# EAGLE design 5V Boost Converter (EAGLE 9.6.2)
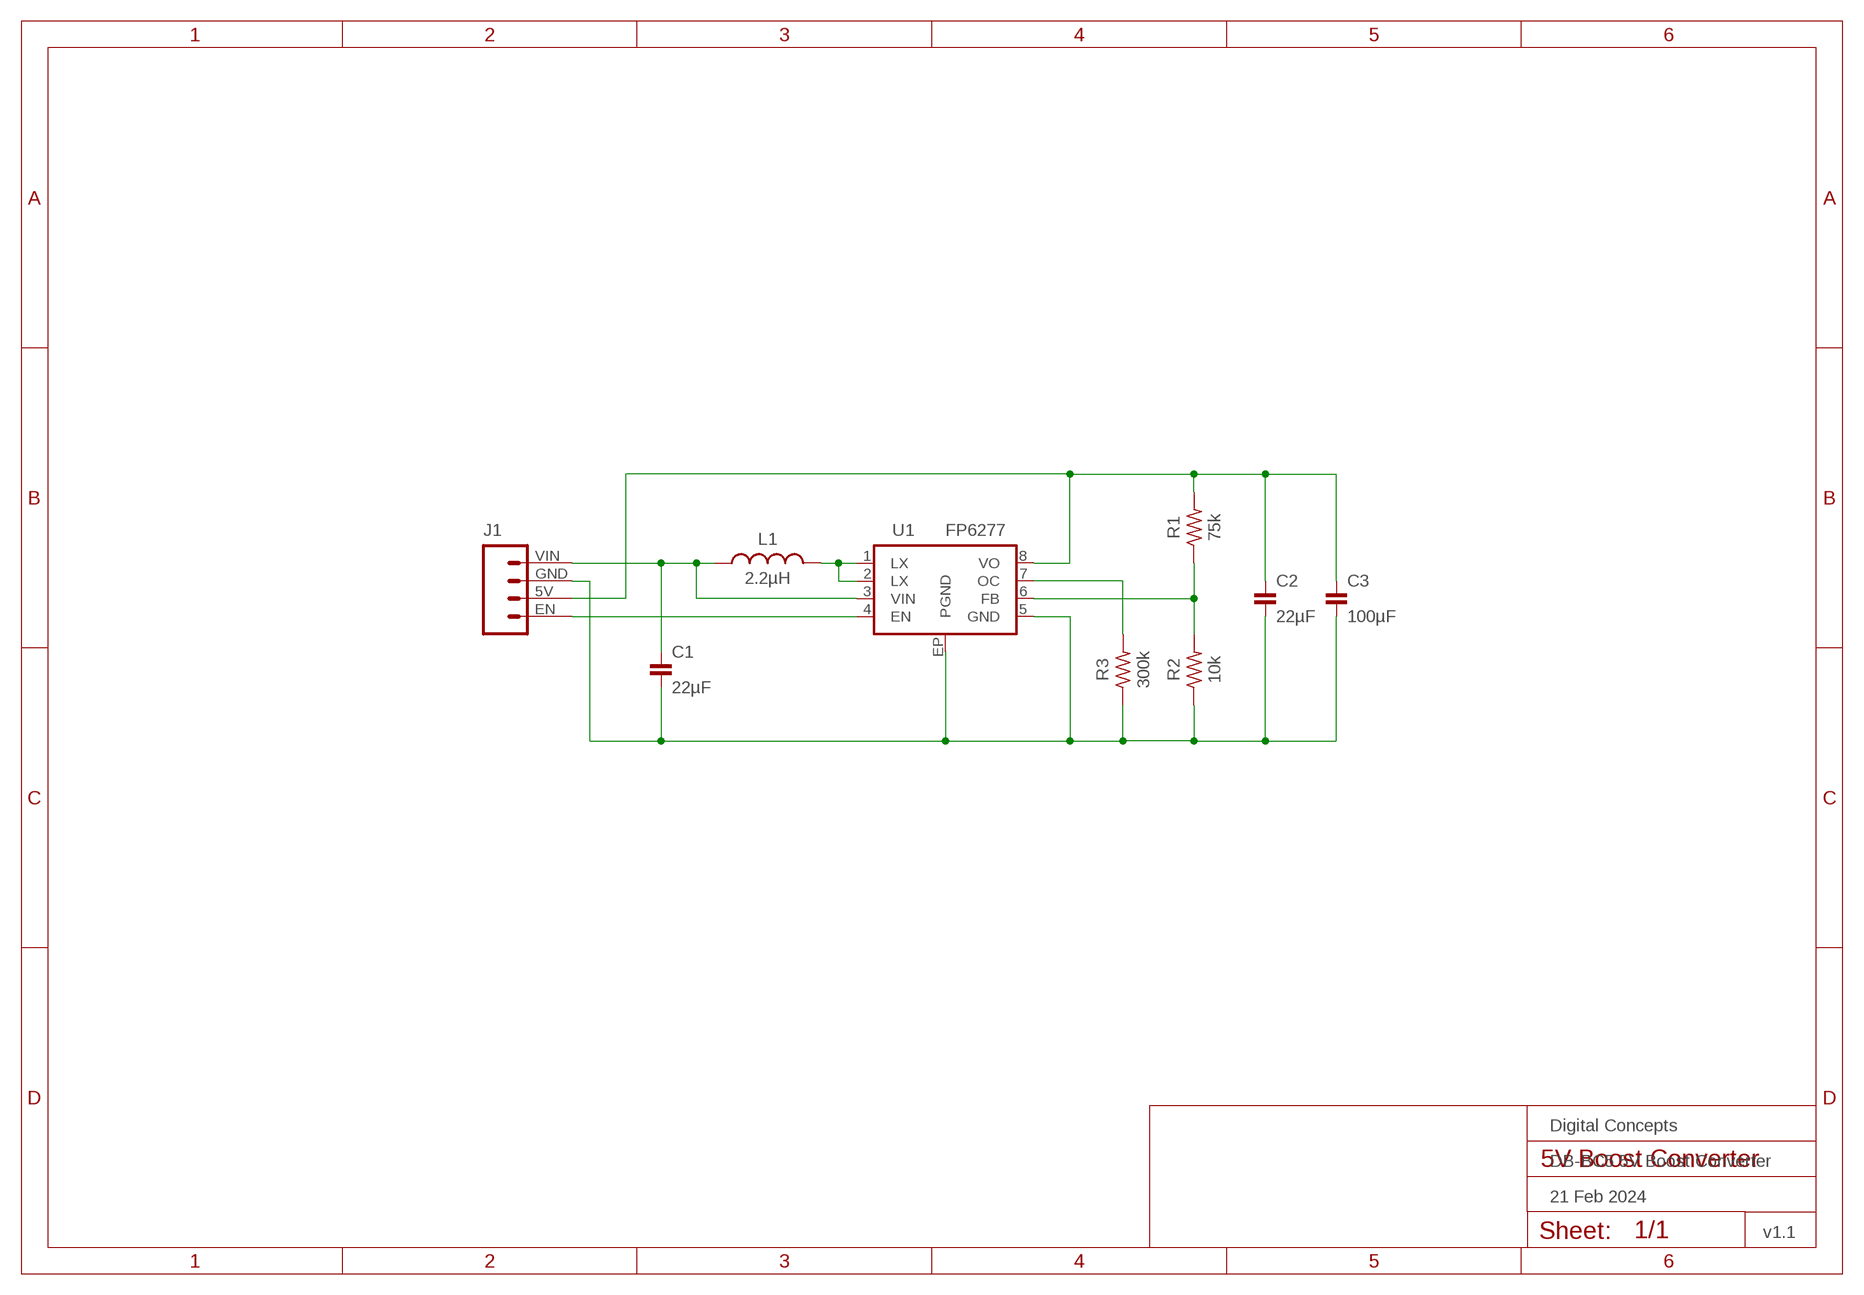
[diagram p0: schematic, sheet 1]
FRAME2 (FRAME-A4L-LOC): DATE: 21 Feb 2024; OWNER: Digital Concepts; TITLE: DB-BC5 5V Boost Converter; VERSION: v1.1

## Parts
C1  22µF  CAPACITOR-0805  [C0805]
C2  22µF  CAPACITOR-0805  [C0805]
C3  100µF  CAPACITOR-1206  [C1206]
J1  HEADER-1X4-FP6277  [CONN_04-FP6277]
L1  2.2µH  INDUCTOR-LQM2HPN2R2MG0L  [L1008]
R1  75k  RESISTORR0805  [R0805]
R2  10k  RESISTORR0805  [R0805]
R3  300k  RESISTORR0805  [R0805]
U1  FP6277  [SOP-8(EP)]

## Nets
5V: C2.1 C3.1 J1.5V R1.2 U1.8(VO)
EN: J1.EN U1.4(EN)
GND: C1.2 C2.2 C3.2 J1.GND R2.1 R3.1 U1.5(GND) U1.EP(PGND)
N$2: L1.P$1 U1.1(LX) U1.2(LX)
N$3: R1.1 R2.2 U1.6(FB)
N$5: R3.2 U1.7(OC)
VIN: C1.1 J1.VIN L1.P$2 U1.3(VIN)

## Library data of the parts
C1 C2 = digitalconcepts:CAPACITOR-0805: 0805 Capacitor
C3 = digitalconcepts:CAPACITOR-1206: 1206 Capacitor
J1 = digitalconcepts:HEADER-1X4-FP6277: FP6277 4-Pin Header
L1 = digitalconcepts:INDUCTOR-LQM2HPN2R2MG0L: LQM2HPN2R2MG0L
R1-R3 = digitalconcepts:RESISTOR: Resistor; SPICEPREFIX: R
U1 = digitalconcepts:FP6277: FP6277 Boost Controller

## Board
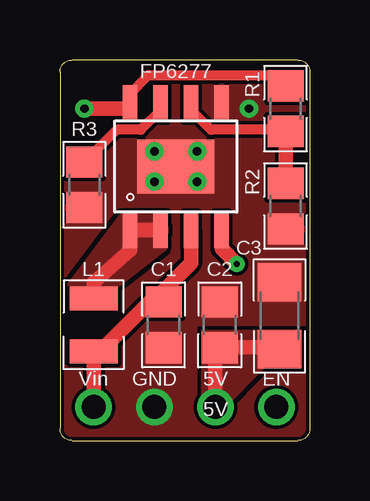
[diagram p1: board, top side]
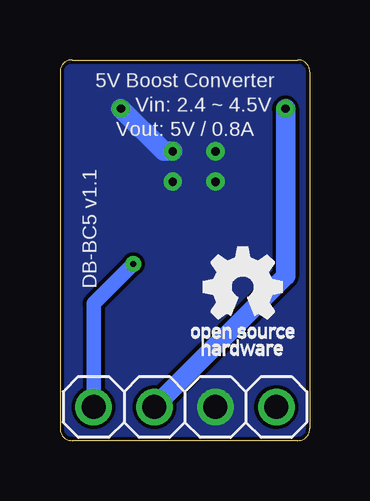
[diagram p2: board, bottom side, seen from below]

Size 10.41 x 15.88 mm. Coordinates in mm from the lower left corner, seen from the top.
Outline: 9.91,15.88 arc-90 10.41,15.37 10.41,0.51 arc-90 9.91,0 0.51,0 arc-90 0,0.51 0,15.37 arc-90 0.51,15.88 9.91,15.88
Copper layers (1*16): Top 0.035mm / dielectric 1.5mm / Bottom 0.035mm
Design rules "default *": minimum track width 6mil, minimum drill 0.15mm, track to track 6mil, track to pad 6mil, pad to pad 6mil, via to via 6mil, smd to smd 6mil, copper to edge 6mil, drill to drill 6mil, minimum pad ring 10mil, minimum via ring 8mil, stop-mask expansion 4mil, vias tented up to drill 0mil, thermal gap 0mil

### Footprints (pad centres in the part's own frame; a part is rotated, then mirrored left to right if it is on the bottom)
C0805 = smd 1.3 x 1.5: 1 -0.95,0; 2 0.95,0
C1206 = smd 1.6 x 1.8: 1 -1.4,0; 2 1.4,0
CONN_04-FP6277 = drill 1 pad 1.524: 5V 2.54,0; EN 0,0; GND 5.08,0; VIN 7.62,0
L1008 = smd 1 x 2: P$1 -1.1,0; P$2 1.1,0
R0805 = smd 1.3 x 1.5: 1 -0.95,0; 2 0.95,0
SOP-8(EP) = smd 0.6 x 1.5: 1 -1.905,-2.64; 2 -0.635,-2.64; 3 0.635,-2.64; 4 1.905,-2.64; 5 1.905,2.64; 6 0.635,2.64; 7 -0.635,2.64; 8 -1.905,2.64 | smd 3.2 x 2.26: EP 0,0

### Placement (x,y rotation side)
C1  4.32,4.83 270 top
C2  6.65,4.83 90 top
C3  9.14,5.21 90 top
J1  9.02,1.4 0 bottom
L1  1.4,4.83 270 top
R1  9.4,13.84 90 top
R2  9.4,9.78 90 top
R3  1.02,10.67 90 top
U1  4.83,11.43 0 top

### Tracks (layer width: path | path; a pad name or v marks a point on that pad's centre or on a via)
5V  (via drill 0.35)
  Top 0.406: U1.8 2.92,14.48 3.68,15.24 9.4,15.24 R1.2 | C3.1 9.13,3.88
  Top 0.61: 9.13,3.88 C2.1 6.48,3.75 J1.5V | U1.8 2.69,13.84 v1.02,13.84
  Bottom 0.813: v1.02,13.84 1.02,6.86 J1.5V
  pour Top (no thermals): 5.92,4.6 10.03,4.6 10.03,3.02 8.48,3.02 6.73,1.27 6.25,1.27 5.92,1.49
EN  (via drill 0.25 pad 0.65)
  Top 0.61: v7.37,7.37 6.73,8 U1.4
  Bottom 0.61: v7.37,7.37 9.02,5.71 J1.EN
GND  (via drill 0.35)
  Bottom 0.813: v7.87,13.84 6.1,12.06 v5.71,12.06
  other vias: 3.94,12.06 5.71,10.79 3.94,10.79
  pour Top (rank 5): -0.51,16.38 10.92,16.38 10.92,-0.51 -0.51,-0.51
  pour Bottom: -0.25,16.13 10.67,16.13 10.67,-0.25 -0.25,-0.25
N$2
  Top 0.61: U1.2 U1.1 2.92,7.94 1.4,6.59 L1.P$1
  pour Top: 0.33,6.48 2.62,9.53 4.5,9.53 4.5,8.03 2.49,6.48
N$3
  Top 0.406: U1.6 5.46,13.79 6.28,12.96 9.39,12.96 R1.1
  Top 0.61: R1.1 R2.2
N$5
  Top 0.406: R3.2 2.36,12.96 3.37,12.96 4.19,13.79 U1.7
VIN
  Top 0.61: U1.3 5.46,7.4 4.32,6.26 C1.1 3.75,5.78 1.5,3.53 L1.P$2 J1.VIN

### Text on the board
bPlace: 5V Boost Converter | Vin: 2.4 ~ 4.5V | Vout: 5V / 0.8A | DB-BC5 v1.1
tNames: Vin | GND | 5V | EN | 5V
